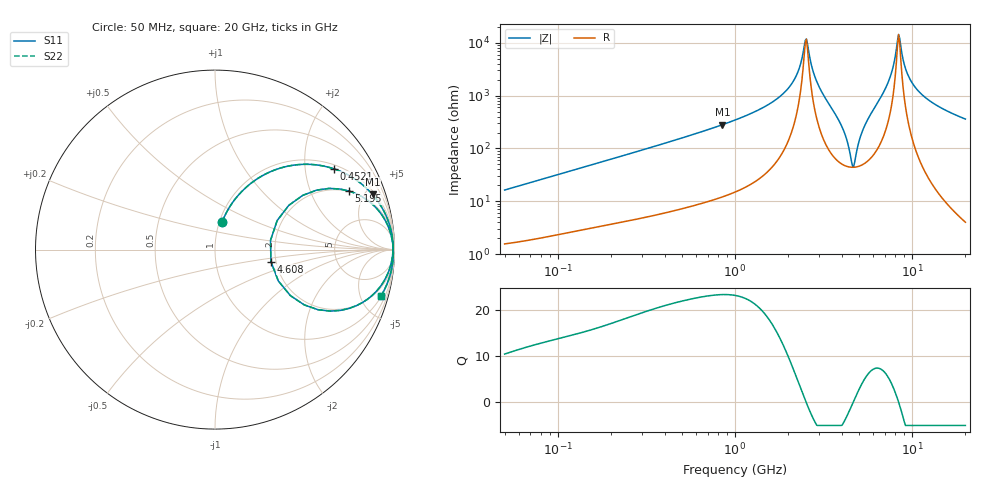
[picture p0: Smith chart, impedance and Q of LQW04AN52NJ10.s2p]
!Murata Part Number: LQW04AN52NJ10
!These Parameters are Measured in Series Mode Connection
!  o--[Z]--o
!Port1  Port2
!  o-------o
!Freq. Start=50[MHz] Stop=20[GHz], 401[Steps]
# Hz S RI R 50
!Freq.(Hz) S11(Real) S11(Imag) S21(Real) S21(Imag) S12(Real) S12(Imag) S22(Real) S22(Imag)
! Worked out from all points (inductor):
!   401 points, 50 MHz to 20 GHz, reference 50 ohm
!   read as one part in series: L = 51.4 nH near 51.52 MHz
!   highest Q = 23.3 at 848.1 MHz (marker M1), where L = 52.7 nH
!   self-resonance near 2.494 GHz
!   S11 on the Smith chart (normalised r, x): 50 MHz: 1.03, +0.32; 452.1 MHz: 1.13, +2.83; 4.608 GHz: 1.88, -0.28; 5.195 GHz: 1.97, +3.82; 20 GHz: 1.08, -7.20
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5e7  0.0398 0.1534  0.9602 -0.1534  0.9602 -0.1534  0.0398 0.1534
1.364002e8  0.1733 0.3468  0.8267 -0.3468  0.8267 -0.3468  0.1733 0.3468
3.721004e8  0.5712 0.4712  0.4288 -0.4712  0.4288 -0.4712  0.5712 0.4712
4.520922e8  0.6606 0.4508  0.3394 -0.4508  0.3394 -0.4508  0.6606 0.4508
8.480927e8  0.8776 0.307  0.1224 -0.307  0.1224 -0.307  0.8776 0.307
1e9  0.9128 0.2613  0.0872 -0.2613  0.0872 -0.2613  0.9128 0.2613
1.932977e9  0.9862 0.0802  0.0138 -0.0802  0.0138 -0.0802  0.9862 0.0802
2.245319e9  0.9912 0.0369  0.00882 -0.0369  0.00882 -0.0369  0.9912 0.0369
2.493527e9  0.9919 0.00381  0.00813 -0.00381  0.00813 -0.00381  0.9919 0.00381
2.569357e9  0.9915 -0.00635  0.00847 0.00635  0.00847 0.00635  0.9915 -0.00635
2.728004e9  0.9899 -0.028  0.0101 0.028  0.0101 0.028  0.9899 -0.028
3.029571e9  0.9827 -0.072  0.0173 0.072  0.0173 0.072  0.9827 -0.072
3.850025e9  0.8881 -0.2436  0.1119 0.2436  0.1119 0.2436  0.8881 -0.2436
4.34015e9  0.5736 -0.3347  0.4264 0.3347  0.4264 0.3347  0.5736 -0.3347
4.608136e9  0.3117 -0.0668  0.6883 0.0668  0.6883 0.0668  0.3117 -0.0668
4.89267e9  0.4889 0.3023  0.5111 -0.3023  0.5111 -0.3023  0.4889 0.3023
5.194772e9  0.7463 0.3265  0.2537 -0.3265  0.2537 -0.3265  0.7463 0.3265
7.442007e9  0.9883 0.0468  0.0117 -0.0468  0.0117 -0.0468  0.9883 0.0468
8.389408e9  0.9931 0.000422  0.00688 -0.000422  0.00688 -0.000422  0.9931 0.000422
9.457416e9  0.993 -0.0391  0.007 0.0391  0.007 0.0391  0.993 -0.0391
1.066139e10  0.9897 -0.0752  0.0103 0.0752  0.0103 0.0752  0.9897 -0.0752
2e10  0.9259 -0.2564  0.0741 0.2564  0.0741 0.2564  0.9259 -0.2564
